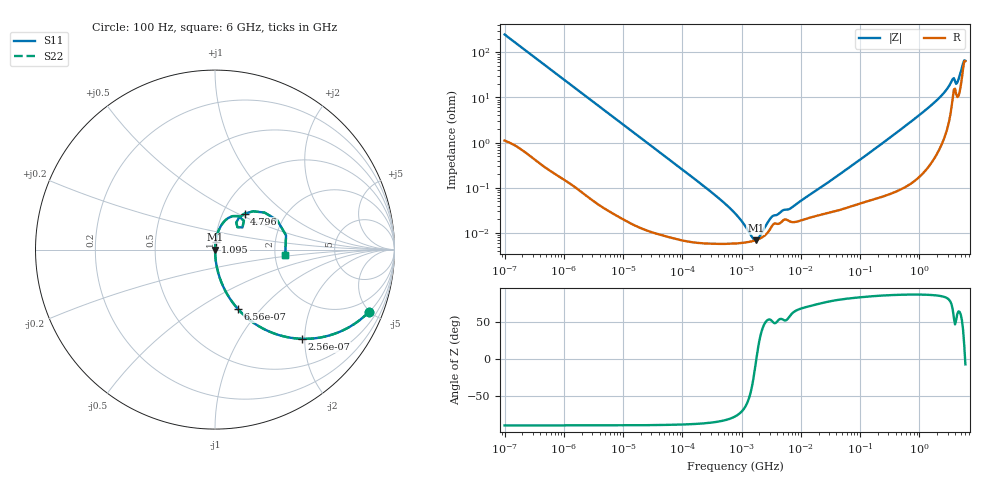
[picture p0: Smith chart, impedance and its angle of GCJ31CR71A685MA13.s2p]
!Murata Part Number: GCJ31CR71A685MA13
!These Parameters are Measured in Series Mode Connection
!Data Generated on Mar 13, 2026
!  o--ll--o
!Port1  Port2
!  o------o
!Operation Temp=25[degC], DC Bias Voltage=0[V]
!Freq. Start=100[Hz] Stop=6[GHz] 401[Steps]
# Hz S RI R 50
!Freq.(Hz) S11(Real) S11(Imag) S21(Real) S21(Imag) S12(Real) S12(Imag) S22(Real) S22(Imag)
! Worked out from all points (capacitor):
!   401 points, 100 Hz to 6 GHz, reference 50 ohm
!   read as one part in series: C = 6.41 uF near 109 Hz
!   lowest |Z| = 6.96 mohm at 1.734 MHz (marker M1)
!   series resonance near 1.774 MHz, so ESL is about 1.3 nH
!   S11 on the Smith chart (normalised r, x): 100 Hz: 1.02, -4.96; 256 Hz: 1.01, -1.94; 656 Hz: 1.00, -0.76; 1.095 GHz: 1.00, +0.09; 4.796 GHz: 1.26, +0.54; 6 GHz: 2.28, -0.16
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100  0.8589 -0.3459  0.1411 0.3459  0.1411 0.3459  0.8589 -0.3459
256  0.4857 -0.4971  0.5143 0.4971  0.5143 0.4971  0.4857 -0.4971
656  0.128 -0.3312  0.872 0.3312  0.872 0.3312  0.128 -0.3312
2008  0.0161 -0.1227  0.9839 0.1227  0.9839 0.1227  0.0161 -0.1227
6433  0.00181 -0.0391  0.9982 0.0391  0.9982 0.0391  0.00181 -0.0391
40335  0.000133 -0.00628  0.9999 0.00628  0.9999 0.00628  0.000133 -0.00628
316350  5.83e-05 -0.000781  0.9999 0.000781  0.9999 0.000781  5.83e-05 -0.000781
774597  5.86e-05 -0.000267  0.9999 0.000267  0.9999 0.000267  5.86e-05 -0.000267
1325623  6.34e-05 -8.57e-05  0.9999 8.57e-05  0.9999 8.57e-05  6.34e-05 -8.57e-05
1734173  6.93e-05 -6.6e-06  0.9999 6.6e-06  0.9999 6.6e-06  6.93e-05 -6.6e-06
2169299  7.86e-05 5.99e-05  0.9999 -5.99e-05  0.9999 -5.99e-05  7.86e-05 5.99e-05
3394479  0.000154 0.000184  0.9998 -0.000184  0.9998 -0.000184  0.000154 0.000184
6644369  0.000179 0.0003  0.9998 -0.0003  0.9998 -0.0003  0.000179 0.0003
1.555665e7  0.000227 0.000728  0.9998 -0.000728  0.9998 -0.000728  0.000227 0.000728
3.124326e8  0.000878 0.0126  0.9991 -0.0126  0.9991 -0.0126  0.000878 0.0126
1.094528e9  0.00393 0.0445  0.9961 -0.0445  0.9961 -0.0445  0.00393 0.0445
2.802721e9  0.0342 0.1341  0.9658 -0.1341  0.9658 -0.1341  0.0342 0.1341
3.505958e9  0.0969 0.1864  0.9031 -0.1864  0.9031 -0.1864  0.0969 0.1864
4.385646e9  0.1186 0.1508  0.8814 -0.1508  0.8814 -0.1508  0.1186 0.1508
4.796499e9  0.1651 0.2008  0.8349 -0.2008  0.8349 -0.2008  0.1651 0.2008
5.245841e9  0.2755 0.2064  0.7245 -0.2064  0.7245 -0.2064  0.2755 0.2064
6e9  0.3914 -0.0291  0.6086 0.0291  0.6086 0.0291  0.3914 -0.0291
